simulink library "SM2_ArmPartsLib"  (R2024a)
settings: Solver=ode45  StartTime=0.0  StopTime=10.0  RelTol=1e-3  EnableMultiTasking=on
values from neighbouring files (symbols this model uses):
  m = v*BEAM.rho    [FlexBeamModelConstruct2.m]    (also in FlexBeamModelConstruct3.m = BEAM.rho*v; FlexBeam_1D_Construct.m = REF.m/REF.l*a.*(linspace(1-OPT.MassBiais+1e-6,1+OPT.MassBiai; FlexBeam_3D_Construct.m = REF.m/REF.l*a.*(linspace(1-OPT.MassBiais+1e-6,1+OPT.MassBiai; FreeFlexBeam_3D_Construct.m = REF.m/REF.l*a.*tmp2)
  N = D(1)+(H4^2+H3^2)/H2^2-(E(1)*H4+F(1)*H3)/H2    [MGD.m]    (also in MGD2.m)
  s = -sign(imag(KGZ_fr_tmp))    [LinprogReguliOptimFunc_1.m]    (also in LinprogReguliOptimFunc_2.m; LinprogReguliOptimFunc_1 - Copie.m)
  X = cos(phi(i))*x+sin(phi(i))*y    [MGI.m]
  Y = fft(y(:,i),NFFT)/L    [fft_bis.m]    (also in MGI.m = -sin(phi(i))*x+cos(phi(i))*y)
  Z = z    [MGI.m]
undefined symbols (not defined in the file or in its folder): deg, kg, rad, SimParam
libraries: $bdroot x38, sm_lib x32
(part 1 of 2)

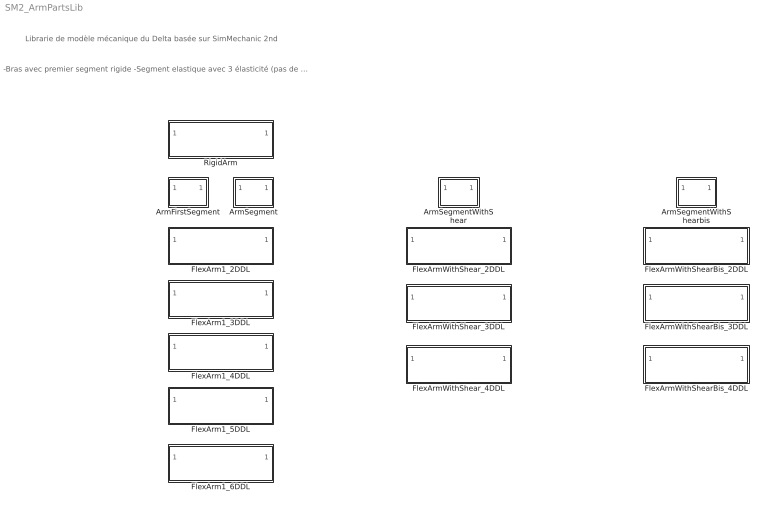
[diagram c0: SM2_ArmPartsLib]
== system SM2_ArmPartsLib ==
  note: -Bras avec premier segment rigide -Segment elastique avec 3 élasticité (pas de cisaillement)
  note: Librarie de modèle mécanique du Delta basée sur SimMechanic 2nd
  ArmFirstSegment : Subsystem  mask{ID=1}
      mask prompts: ID "Segment ID"
  ArmSegment : Subsystem  mask{ID=2}
      mask prompts: ID "Segment ID"
  ArmSegmentWithShear : Subsystem  mask{ID=1}
      mask prompts: ID "Segment ID"
  ArmSegmentWithShearbis : Subsystem  mask{ID=1}
      mask prompts: ID "Segment ID"
  FlexArm1_2DDL : Subsystem  InitFcn=SimParam.Arm = flexArm1_paramInitFnc(RawParam,2,1);  VariantControl=armVarFlex1_2ddl
  FlexArm1_3DDL : Subsystem  InitFcn=SimParam.Arm = flexArm1_paramInitFnc(RawParam,3,1);  VariantControl=armVarFlex1_3ddl
  FlexArm1_4DDL : Subsystem  InitFcn=SimParam.Arm = flexArm1_paramInitFnc(RawParam,4,1);  VariantControl=armVarFlex1_4ddl
  FlexArm1_5DDL : Subsystem  InitFcn=SimParam.Arm = flexArm1_paramInitFnc(RawParam,5,1);  VariantControl=armVarFlex1_4ddl
  FlexArm1_6DDL : Subsystem  InitFcn=SimParam.Arm = flexArm1_paramInitFnc(RawParam,6,1);  VariantControl=armVarFlex1_4ddl
  FlexArmWithShearBis_2DDL : Subsystem  InitFcn=SimParam.Arm = flexArm1_paramInitFnc(RawParam,2,2);  VariantControl=armVarFlex1_2ddl
  FlexArmWithShearBis_3DDL : Subsystem  InitFcn=SimParam.Arm = flexArm1_paramInitFnc(RawParam,3,2);  VariantControl=armVarFlex1_2ddl
  FlexArmWithShearBis_4DDL : Subsystem  InitFcn=SimParam.Arm = flexArm1_paramInitFnc(RawParam,4,2);  VariantControl=armVarFlex1_2ddl
  FlexArmWithShear_2DDL : Subsystem  InitFcn=SimParam.Arm = flexArm1_paramInitFnc(RawParam,2,2);  VariantControl=armVarFlex1_2ddl
  FlexArmWithShear_3DDL : Subsystem  InitFcn=SimParam.Arm = flexArm1_paramInitFnc(RawParam,3,2);  VariantControl=armVarFlex1_2ddl
  FlexArmWithShear_4DDL : Subsystem  InitFcn=SimParam.Arm = flexArm1_paramInitFnc(RawParam,4,2);  VariantControl=armVarFlex1_2ddl
  RigidArm : Subsystem  InitFcn=SimParam.Arm=RigidArm_paramInitFnc(RawParam,0);  VariantControl=armVarDefault

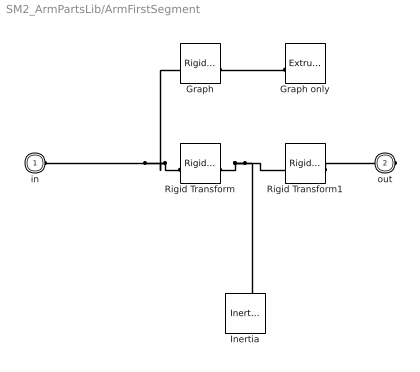
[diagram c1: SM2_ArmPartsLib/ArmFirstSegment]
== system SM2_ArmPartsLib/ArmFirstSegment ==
  Graph : sm_lib/Frames and Transforms/Rigid Transform  RotationMethod=AlignedAxes  FollAlignAxisA=+Z  BaseAlignAxisA=+X  FollAlignAxisB=+Y  BaseAlignAxisB=+Z  RotationStandardAxis=+Z  RotationAngle=0  RotationAngleUnits=deg  RotationArbitraryAxis=[0 0 1]  RotationSequenceAxes=FollowerAxes  RotationSequence=XYX  RotationSequenceAngles=[0 0 0]  RotationSequenceAnglesUnits=deg  RotationMatrix=[1 0 0;0 1 0;0 0 1]  Quaternion=[1 0 0 0]  TranslationMethod=Cartesian  TranslationCartesianOffset=[(SimParam.Arm.l(1,ID)+SimParam.Arm.l(2,ID))/2 0 0]  TranslationCartesianOffsetUnits=m  TranslationStandardAxis=+Z  TranslationStandardOffset=0  TranslationStandardOffsetUnits=m  TranslationROffset=0  TranslationROffsetUnits=m  TranslationThetaOffset=0  TranslationThetaOffsetUnits=deg  TranslationZOffset=0  TranslationZOffsetUnits=m
  Graph only : sm_lib/Body Elements/Extruded Solid  ExtrusionType=General  PolygonNumSides=3  PolygonOuterRadius=1  PolygonOuterRadiusUnits=m  ExportEntireGeometry=off  ExtrusionCrossSection=0.01.*[1 1; -1 1; -1 -1; 1 -1]  ExtrusionCrossSectionUnits=m  ExportConvexHullGeometry=off  ExtrusionLength=SimParam.Arm.l(1,ID)+SimParam.Arm.l(2,ID)  ExtrusionLengthUnits=m  InertiaType=PointMass  BasedOnType=Density  Density=1000  DensityUnits=kg/(m^3)  Mass=0  MassUnits=kg  CenterOfMass=[0 0 0]  CenterOfMassUnits=m  MomentsOfInertia=[0 0 0]  MomentsOfInertiaUnits=kg*m^2  ProductsOfInertia=[0 0 0]  ProductsOfInertiaUnits=kg*m^2  GraphicType=FromGeometry  MarkerShape=Sphere  MarkerSize=10  GraphicVisPropType=SimpleVisualProperties  GraphicDiffuseColor=[0.5 0.5 0.5]  GraphicOpacity=1.0  GraphicSpecularColor=[0.5 0.5 0.5 1.0]  GraphicAmbientColor=[0.15 0.15 0.15 1.0]  GraphicEmissiveColor=[0.0 0.0 0.0 1.0]  GraphicShininess=75  DoExposeReferenceFrame=on  SerializedFrames=<Frames/>
  Inertia : sm_lib/Body Elements/Inertia  InertiaType=Custom  Mass=SimParam.Arm.m(ID)  MassUnits=kg  CenterOfMass=[0 0 0]  CenterOfMassUnits=m  MomentsOfInertia=SimParam.Arm.I(:,ID)'  MomentsOfInertiaUnits=kg*m^2  ProductsOfInertia=[0 0 0]  ProductsOfInertiaUnits=kg*m^2  GraphicType=Marker  MarkerShape=Inertia  MarkerSize=20  GraphicVisPropType=SimpleVisualProperties  GraphicDiffuseColor=[0.5 0.5 0.5]  GraphicOpacity=1  GraphicSpecularColor=[0.5 0.5 0.5 1.0]  GraphicAmbientColor=[0.15 0.15 0.15 1.0]  GraphicEmissiveColor=[0.0 0.0 0.0 1.0]  GraphicShininess=75
  Rigid Transform : sm_lib/Frames and Transforms/Rigid Transform  RotationMethod=None  FollAlignAxisA=+X  BaseAlignAxisA=+Y  FollAlignAxisB=+Y  BaseAlignAxisB=+Z  RotationStandardAxis=+Z  RotationAngle=0  RotationAngleUnits=deg  RotationArbitraryAxis=[0 0 1]  RotationSequenceAxes=FollowerAxes  RotationSequence=XYX  RotationSequenceAngles=[0 0 0]  RotationSequenceAnglesUnits=deg  RotationMatrix=[1 0 0;0 1 0;0 0 1]  Quaternion=[1 0 0 0]  TranslationMethod=Cartesian  TranslationCartesianOffset=[SimParam.Arm.l(1,ID) 0 0]  TranslationCartesianOffsetUnits=m  TranslationStandardAxis=+Z  TranslationStandardOffset=0  TranslationStandardOffsetUnits=m  TranslationROffset=0  TranslationROffsetUnits=m  TranslationThetaOffset=0  TranslationThetaOffsetUnits=deg  TranslationZOffset=0  TranslationZOffsetUnits=m
  Rigid Transform1 : sm_lib/Frames and Transforms/Rigid Transform  RotationMethod=None  FollAlignAxisA=+X  BaseAlignAxisA=+Y  FollAlignAxisB=+Y  BaseAlignAxisB=+Z  RotationStandardAxis=+Z  RotationAngle=0  RotationAngleUnits=deg  RotationArbitraryAxis=[0 0 1]  RotationSequenceAxes=FollowerAxes  RotationSequence=XYX  RotationSequenceAngles=[0 0 0]  RotationSequenceAnglesUnits=deg  RotationMatrix=[1 0 0;0 1 0;0 0 1]  Quaternion=[1 0 0 0]  TranslationMethod=Cartesian  TranslationCartesianOffset=[SimParam.Arm.l(2,ID) 0 0]  TranslationCartesianOffsetUnits=m  TranslationStandardAxis=+Z  TranslationStandardOffset=0  TranslationStandardOffsetUnits=m  TranslationROffset=0  TranslationROffsetUnits=m  TranslationThetaOffset=0  TranslationThetaOffsetUnits=deg  TranslationZOffset=0  TranslationZOffsetUnits=m
  in : PMIOPort  Side=Left
  out : PMIOPort  Port=2  Side=Right
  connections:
  Rigid Transform/RConn1 -- Rigid Transform1/LConn1 -- Inertia/RConn1
  Rigid Transform1/RConn1 -- out/RConn1
  Rigid Transform/LConn1 -- in/RConn1 -- Graph/LConn1
  Graph only/RConn1 -- Graph/RConn1

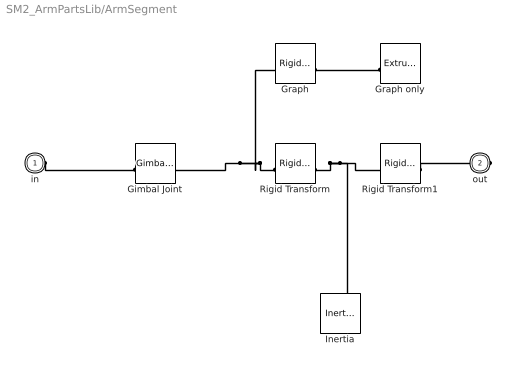
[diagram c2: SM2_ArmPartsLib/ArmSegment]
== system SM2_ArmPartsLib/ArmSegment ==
  Gimbal Joint : sm_lib/Joints/Gimbal Joint  JointMode=Normal  CompositeWrenchDir=FollowerOnBase  CompositeWrenchFrame=BaseFrame  SenseConstraintForce=off  SenseConstraintTorque=off  SenseTotalForce=off  SenseTotalTorque=off  RxPositionTargetSpecify=on  RxPositionTargetPriority=High  RxPositionTargetValue=0  RxPositionTargetValueUnits=rad  RxVelocityTargetSpecify=on  RxVelocityTargetPriority=High  RxVelocityTargetValue=0  RxVelocityTargetValueUnits=rad/s  RxEquilibriumPosition=0  RxEquilibriumPositionUnits=rad  RxSpringStiffness=SimParam.Arm.k(1,ID)  RxSpringStiffnessUnits=N*m/rad  RxDampingCoefficient=SimParam.Arm.c(1,ID)  RxDampingCoefficientUnits=N*m/(rad/s)  RxLowerLimitSpecify=off  RxLowerLimitBound=-90  RxLowerLimitBoundUnits=deg  RxLowerLimitStiffness=1e4  RxLowerLimitStiffnessUnits=N*m/deg  RxLowerLimitDamping=10  RxLowerLimitDampingUnits=N*m/(deg/s)  RxLowerLimitTransitionRegionWidth=0.1  RxLowerLimitTransitionRegionWidthUnits=deg  RxUpperLimitSpecify=off  RxUpperLimitBound=90  RxUpperLimitBoundUnits=deg  RxUpperLimitStiffness=1e4  RxUpperLimitStiffnessUnits=N*m/deg  RxUpperLimitDamping=10  RxUpperLimitDampingUnits=N*m/(deg/s)  RxUpperLimitTransitionRegionWidth=0.1  RxUpperLimitTransitionRegionWidthUnits=deg  RxTorqueActuationMode=NoTorque  RxMotionActuationMode=ComputedMotion  RxSensePosition=off  RxSenseVelocity=off  RxSenseAcceleration=off  RxSenseTorqueForce=off  RxSenseLowerLimitTorqueForce=off  RxSenseUpperLimitTorqueForce=off  RyPositionTargetSpecify=on  RyPositionTargetPriority=High  RyPositionTargetValue=0  RyPositionTargetValueUnits=rad  RyVelocityTargetSpecify=on  RyVelocityTargetPriority=High  RyVelocityTargetValue=0  RyVelocityTargetValueUnits=rad/s  RyEquilibriumPosition=0  RyEquilibriumPositionUnits=rad  RySpringStiffness=SimParam.Arm.k(2,ID)  RySpringStiffnessUnits=N*m/rad  RyDampingCoefficient=SimParam.Arm.c(2,ID)  RyDampingCoefficientUnits=N*m/(rad/s)  RyLowerLimitSpecify=off  RyLowerLimitBound=-90  RyLowerLimitBoundUnits=deg  RyLowerLimitStiffness=1e4  RyLowerLimitStiffnessUnits=N*m/deg  RyLowerLimitDamping=10  RyLowerLimitDampingUnits=N*m/(deg/s)  RyLowerLimitTransitionRegionWidth=0.1  RyLowerLimitTransitionRegionWidthUnits=deg  RyUpperLimitSpecify=off  RyUpperLimitBound=90  RyUpperLimitBoundUnits=deg  RyUpperLimitStiffness=1e4  RyUpperLimitStiffnessUnits=N*m/deg  RyUpperLimitDamping=10  RyUpperLimitDampingUnits=N*m/(deg/s)  RyUpperLimitTransitionRegionWidth=0.1  RyUpperLimitTransitionRegionWidthUnits=deg  RyTorqueActuationMode=NoTorque  RyMotionActuationMode=ComputedMotion  RySensePosition=off  RySenseVelocity=off  RySenseAcceleration=off  RySenseTorqueForce=off  RySenseLowerLimitTorqueForce=off  RySenseUpperLimitTorqueForce=off  RzPositionTargetSpecify=on  RzPositionTargetPriority=High  RzPositionTargetValue=0  RzPositionTargetValueUnits=rad  RzVelocityTargetSpecify=on  RzVelocityTargetPriority=High  RzVelocityTargetValue=0  RzVelocityTargetValueUnits=rad/s  RzEquilibriumPosition=0  RzEquilibriumPositionUnits=rad  RzSpringStiffness=SimParam.Arm.k(3,ID)  RzSpringStiffnessUnits=N*m/rad  RzDampingCoefficient=SimParam.Arm.c(3,ID)  RzDampingCoefficientUnits=N*m/(rad/s)  RzLowerLimitSpecify=off  RzLowerLimitBound=-90  RzLowerLimitBoundUnits=deg  RzLowerLimitStiffness=1e4  RzLowerLimitStiffnessUnits=N*m/deg  RzLowerLimitDamping=10  RzLowerLimitDampingUnits=N*m/(deg/s)  RzLowerLimitTransitionRegionWidth=0.1  RzLowerLimitTransitionRegionWidthUnits=deg  RzUpperLimitSpecify=off  RzUpperLimitBound=90  RzUpperLimitBoundUnits=deg  RzUpperLimitStiffness=1e4  RzUpperLimitStiffnessUnits=N*m/deg  RzUpperLimitDamping=10  RzUpperLimitDampingUnits=N*m/(deg/s)  RzUpperLimitTransitionRegionWidth=0.1  RzUpperLimitTransitionRegionWidthUnits=deg  RzTorqueActuationMode=NoTorque  RzMotionActuationMode=ComputedMotion  RzSensePosition=off  RzSenseVelocity=off  RzSenseAcceleration=off  RzSenseTorqueForce=off  RzSenseLowerLimitTorqueForce=off  RzSenseUpperLimitTorqueForce=off
  Graph : sm_lib/Frames and Transforms/Rigid Transform  RotationMethod=AlignedAxes  FollAlignAxisA=+Z  BaseAlignAxisA=+X  FollAlignAxisB=+Y  BaseAlignAxisB=+Z  RotationStandardAxis=+Z  RotationAngle=0  RotationAngleUnits=deg  RotationArbitraryAxis=[0 0 1]  RotationSequenceAxes=FollowerAxes  RotationSequence=XYX  RotationSequenceAngles=[0 0 0]  RotationSequenceAnglesUnits=deg  RotationMatrix=[1 0 0;0 1 0;0 0 1]  Quaternion=[1 0 0 0]  TranslationMethod=Cartesian  TranslationCartesianOffset=[(SimParam.Arm.l(1,ID)+SimParam.Arm.l(2,ID))/2 0 0]  TranslationCartesianOffsetUnits=m  TranslationStandardAxis=+Z  TranslationStandardOffset=0  TranslationStandardOffsetUnits=m  TranslationROffset=0  TranslationROffsetUnits=m  TranslationThetaOffset=0  TranslationThetaOffsetUnits=deg  TranslationZOffset=0  TranslationZOffsetUnits=m
  Graph only : sm_lib/Body Elements/Extruded Solid  ExtrusionType=General  PolygonNumSides=3  PolygonOuterRadius=1  PolygonOuterRadiusUnits=m  ExportEntireGeometry=off  ExtrusionCrossSection=0.01.*[1 1; -1 1; -1 -1; 1 -1]  ExtrusionCrossSectionUnits=m  ExportConvexHullGeometry=off  ExtrusionLength=SimParam.Arm.l(1,ID)+SimParam.Arm.l(2,ID)  ExtrusionLengthUnits=m  InertiaType=PointMass  BasedOnType=Density  Density=1000  DensityUnits=kg/(m^3)  Mass=0  MassUnits=kg  CenterOfMass=[0 0 0]  CenterOfMassUnits=m  MomentsOfInertia=[0 0 0]  MomentsOfInertiaUnits=kg*m^2  ProductsOfInertia=[0 0 0]  ProductsOfInertiaUnits=kg*m^2  GraphicType=FromGeometry  MarkerShape=Sphere  MarkerSize=10  GraphicVisPropType=SimpleVisualProperties  GraphicDiffuseColor=[0.5 0.5 0.5]  GraphicOpacity=1.0  GraphicSpecularColor=[0.5 0.5 0.5 1.0]  GraphicAmbientColor=[0.15 0.15 0.15 1.0]  GraphicEmissiveColor=[0.0 0.0 0.0 1.0]  GraphicShininess=75  DoExposeReferenceFrame=on  SerializedFrames=<Frames/>
  Inertia : sm_lib/Body Elements/Inertia  InertiaType=Custom  Mass=SimParam.Arm.m(ID)  MassUnits=kg  CenterOfMass=[0 0 0]  CenterOfMassUnits=m  MomentsOfInertia=SimParam.Arm.I(:,ID)'  MomentsOfInertiaUnits=kg*m^2  ProductsOfInertia=[0 0 0]  ProductsOfInertiaUnits=kg*m^2  GraphicType=Marker  MarkerShape=Inertia  MarkerSize=20  GraphicVisPropType=SimpleVisualProperties  GraphicDiffuseColor=[0.5 0.5 0.5]  GraphicOpacity=1  GraphicSpecularColor=[0.5 0.5 0.5 1.0]  GraphicAmbientColor=[0.15 0.15 0.15 1.0]  GraphicEmissiveColor=[0.0 0.0 0.0 1.0]  GraphicShininess=75
  Rigid Transform : sm_lib/Frames and Transforms/Rigid Transform  RotationMethod=None  FollAlignAxisA=+X  BaseAlignAxisA=+Y  FollAlignAxisB=+Y  BaseAlignAxisB=+Z  RotationStandardAxis=+Z  RotationAngle=0  RotationAngleUnits=deg  RotationArbitraryAxis=[0 0 1]  RotationSequenceAxes=FollowerAxes  RotationSequence=XYX  RotationSequenceAngles=[0 0 0]  RotationSequenceAnglesUnits=deg  RotationMatrix=[1 0 0;0 1 0;0 0 1]  Quaternion=[1 0 0 0]  TranslationMethod=Cartesian  TranslationCartesianOffset=[SimParam.Arm.l(1,ID) 0 0]  TranslationCartesianOffsetUnits=m  TranslationStandardAxis=+Z  TranslationStandardOffset=0  TranslationStandardOffsetUnits=m  TranslationROffset=0  TranslationROffsetUnits=m  TranslationThetaOffset=0  TranslationThetaOffsetUnits=deg  TranslationZOffset=0  TranslationZOffsetUnits=m
  Rigid Transform1 : sm_lib/Frames and Transforms/Rigid Transform  RotationMethod=None  FollAlignAxisA=+X  BaseAlignAxisA=+Y  FollAlignAxisB=+Y  BaseAlignAxisB=+Z  RotationStandardAxis=+Z  RotationAngle=0  RotationAngleUnits=deg  RotationArbitraryAxis=[0 0 1]  RotationSequenceAxes=FollowerAxes  RotationSequence=XYX  RotationSequenceAngles=[0 0 0]  RotationSequenceAnglesUnits=deg  RotationMatrix=[1 0 0;0 1 0;0 0 1]  Quaternion=[1 0 0 0]  TranslationMethod=Cartesian  TranslationCartesianOffset=[SimParam.Arm.l(2,ID) 0 0]  TranslationCartesianOffsetUnits=m  TranslationStandardAxis=+Z  TranslationStandardOffset=0  TranslationStandardOffsetUnits=m  TranslationROffset=0  TranslationROffsetUnits=m  TranslationThetaOffset=0  TranslationThetaOffsetUnits=deg  TranslationZOffset=0  TranslationZOffsetUnits=m
  in : PMIOPort  Side=Left
  out : PMIOPort  Port=2  Side=Right
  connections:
  Rigid Transform/RConn1 -- Rigid Transform1/LConn1 -- Inertia/RConn1
  Rigid Transform/LConn1 -- Gimbal Joint/RConn1 -- Graph/LConn1
  Rigid Transform1/RConn1 -- out/RConn1
  in/RConn1 -- Gimbal Joint/LConn1
  Graph only/RConn1 -- Graph/RConn1

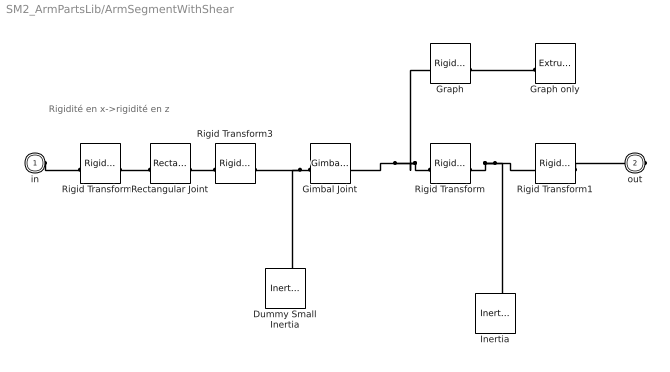
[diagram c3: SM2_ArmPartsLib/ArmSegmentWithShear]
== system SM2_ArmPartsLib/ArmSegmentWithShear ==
  note: Rigidité en x->rigidité en z
  Dummy Small Inertia : sm_lib/Body Elements/Inertia  InertiaType=Custom  Mass=1e-3*SimParam.Arm.m(ID)  MassUnits=kg  CenterOfMass=[0 0 0]  CenterOfMassUnits=m  MomentsOfInertia=1e-4*SimParam.Arm.I(:,ID)'  MomentsOfInertiaUnits=kg*m^2  ProductsOfInertia=[0 0 0]  ProductsOfInertiaUnits=kg*m^2  GraphicType=Marker  MarkerShape=Inertia  MarkerSize=20  GraphicVisPropType=SimpleVisualProperties  GraphicDiffuseColor=[0.5 0.5 0.5]  GraphicOpacity=1  GraphicSpecularColor=[0.5 0.5 0.5 1.0]  GraphicAmbientColor=[0.15 0.15 0.15 1.0]  GraphicEmissiveColor=[0.0 0.0 0.0 1.0]  GraphicShininess=75
  Gimbal Joint : sm_lib/Joints/Gimbal Joint  JointMode=Normal  CompositeWrenchDir=FollowerOnBase  CompositeWrenchFrame=BaseFrame  SenseConstraintForce=off  SenseConstraintTorque=off  SenseTotalForce=off  SenseTotalTorque=off  RxPositionTargetSpecify=on  RxPositionTargetPriority=High  RxPositionTargetValue=0  RxPositionTargetValueUnits=rad  RxVelocityTargetSpecify=on  RxVelocityTargetPriority=High  RxVelocityTargetValue=0  RxVelocityTargetValueUnits=rad/s  RxEquilibriumPosition=0  RxEquilibriumPositionUnits=rad  RxSpringStiffness=SimParam.Arm.k(4,ID)  RxSpringStiffnessUnits=N*m/rad  RxDampingCoefficient=SimParam.Arm.c(4,ID)  RxDampingCoefficientUnits=N*m/(rad/s)  RxLowerLimitSpecify=off  RxLowerLimitBound=-90  RxLowerLimitBoundUnits=deg  RxLowerLimitStiffness=1e4  RxLowerLimitStiffnessUnits=N*m/deg  RxLowerLimitDamping=10  RxLowerLimitDampingUnits=N*m/(deg/s)  RxLowerLimitTransitionRegionWidth=0.1  RxLowerLimitTransitionRegionWidthUnits=deg  RxUpperLimitSpecify=off  RxUpperLimitBound=90  RxUpperLimitBoundUnits=deg  RxUpperLimitStiffness=1e4  RxUpperLimitStiffnessUnits=N*m/deg  RxUpperLimitDamping=10  RxUpperLimitDampingUnits=N*m/(deg/s)  RxUpperLimitTransitionRegionWidth=0.1  RxUpperLimitTransitionRegionWidthUnits=deg  RxTorqueActuationMode=NoTorque  RxMotionActuationMode=ComputedMotion  RxSensePosition=off  RxSenseVelocity=off  RxSenseAcceleration=off  RxSenseTorqueForce=off  RxSenseLowerLimitTorqueForce=off  RxSenseUpperLimitTorqueForce=off  RyPositionTargetSpecify=on  RyPositionTargetPriority=High  RyPositionTargetValue=0  RyPositionTargetValueUnits=rad  RyVelocityTargetSpecify=on  RyVelocityTargetPriority=High  RyVelocityTargetValue=0  RyVelocityTargetValueUnits=rad/s  RyEquilibriumPosition=0  RyEquilibriumPositionUnits=rad  RySpringStiffness=SimParam.Arm.k(5,ID)  RySpringStiffnessUnits=N*m/rad  RyDampingCoefficient=SimParam.Arm.c(5,ID)  RyDampingCoefficientUnits=N*m/(rad/s)  RyLowerLimitSpecify=off  RyLowerLimitBound=-90  RyLowerLimitBoundUnits=deg  RyLowerLimitStiffness=1e4  RyLowerLimitStiffnessUnits=N*m/deg  RyLowerLimitDamping=10  RyLowerLimitDampingUnits=N*m/(deg/s)  RyLowerLimitTransitionRegionWidth=0.1  RyLowerLimitTransitionRegionWidthUnits=deg  RyUpperLimitSpecify=off  RyUpperLimitBound=90  RyUpperLimitBoundUnits=deg  RyUpperLimitStiffness=1e4  RyUpperLimitStiffnessUnits=N*m/deg  RyUpperLimitDamping=10  RyUpperLimitDampingUnits=N*m/(deg/s)  RyUpperLimitTransitionRegionWidth=0.1  RyUpperLimitTransitionRegionWidthUnits=deg  RyTorqueActuationMode=NoTorque  RyMotionActuationMode=ComputedMotion  RySensePosition=off  RySenseVelocity=off  RySenseAcceleration=off  RySenseTorqueForce=off  RySenseLowerLimitTorqueForce=off  RySenseUpperLimitTorqueForce=off  RzPositionTargetSpecify=on  RzPositionTargetPriority=High  RzPositionTargetValue=0  RzPositionTargetValueUnits=rad  RzVelocityTargetSpecify=on  RzVelocityTargetPriority=High  RzVelocityTargetValue=0  RzVelocityTargetValueUnits=rad/s  RzEquilibriumPosition=0  RzEquilibriumPositionUnits=rad  RzSpringStiffness=SimParam.Arm.k(6,ID)  RzSpringStiffnessUnits=N*m/rad  RzDampingCoefficient=SimParam.Arm.c(6,ID)  RzDampingCoefficientUnits=N*m/(rad/s)  RzLowerLimitSpecify=off  RzLowerLimitBound=-90  RzLowerLimitBoundUnits=deg  RzLowerLimitStiffness=1e4  RzLowerLimitStiffnessUnits=N*m/deg  RzLowerLimitDamping=10  RzLowerLimitDampingUnits=N*m/(deg/s)  RzLowerLimitTransitionRegionWidth=0.1  RzLowerLimitTransitionRegionWidthUnits=deg  RzUpperLimitSpecify=off  RzUpperLimitBound=90  RzUpperLimitBoundUnits=deg  RzUpperLimitStiffness=1e4  RzUpperLimitStiffnessUnits=N*m/deg  RzUpperLimitDamping=10  RzUpperLimitDampingUnits=N*m/(deg/s)  RzUpperLimitTransitionRegionWidth=0.1  RzUpperLimitTransitionRegionWidthUnits=deg  RzTorqueActuationMode=NoTorque  RzMotionActuationMode=ComputedMotion  RzSensePosition=off  RzSenseVelocity=off  RzSenseAcceleration=off  RzSenseTorqueForce=off  RzSenseLowerLimitTorqueForce=off  RzSenseUpperLimitTorqueForce=off
  Graph : sm_lib/Frames and Transforms/Rigid Transform  RotationMethod=AlignedAxes  FollAlignAxisA=+Z  BaseAlignAxisA=+X  FollAlignAxisB=+Y  BaseAlignAxisB=+Z  RotationStandardAxis=+Z  RotationAngle=0  RotationAngleUnits=deg  RotationArbitraryAxis=[0 0 1]  RotationSequenceAxes=FollowerAxes  RotationSequence=XYX  RotationSequenceAngles=[0 0 0]  RotationSequenceAnglesUnits=deg  RotationMatrix=[1 0 0;0 1 0;0 0 1]  Quaternion=[1 0 0 0]  TranslationMethod=Cartesian  TranslationCartesianOffset=[(SimParam.Arm.l(1,ID)+SimParam.Arm.l(2,ID))/2 0 0]  TranslationCartesianOffsetUnits=m  TranslationStandardAxis=+Z  TranslationStandardOffset=0  TranslationStandardOffsetUnits=m  TranslationROffset=0  TranslationROffsetUnits=m  TranslationThetaOffset=0  TranslationThetaOffsetUnits=deg  TranslationZOffset=0  TranslationZOffsetUnits=m
  Graph only : sm_lib/Body Elements/Extruded Solid  ExtrusionType=General  PolygonNumSides=3  PolygonOuterRadius=1  PolygonOuterRadiusUnits=m  ExportEntireGeometry=off  ExtrusionCrossSection=0.01.*[1 1; -1 1; -1 -1; 1 -1]  ExtrusionCrossSectionUnits=m  ExportConvexHullGeometry=off  ExtrusionLength=SimParam.Arm.l(1,ID)+SimParam.Arm.l(2,ID)  ExtrusionLengthUnits=m  InertiaType=PointMass  BasedOnType=Density  Density=1000  DensityUnits=kg/(m^3)  Mass=0  MassUnits=kg  CenterOfMass=[0 0 0]  CenterOfMassUnits=m  MomentsOfInertia=[0 0 0]  MomentsOfInertiaUnits=kg*m^2  ProductsOfInertia=[0 0 0]  ProductsOfInertiaUnits=kg*m^2  GraphicType=FromGeometry  MarkerShape=Sphere  MarkerSize=10  GraphicVisPropType=SimpleVisualProperties  GraphicDiffuseColor=[0.5 0.5 0.5]  GraphicOpacity=1.0  GraphicSpecularColor=[0.5 0.5 0.5 1.0]  GraphicAmbientColor=[0.15 0.15 0.15 1.0]  GraphicEmissiveColor=[0.0 0.0 0.0 1.0]  GraphicShininess=75  DoExposeReferenceFrame=on  SerializedFrames=<Frames/>
  Inertia : sm_lib/Body Elements/Inertia  InertiaType=Custom  Mass=SimParam.Arm.m(ID)  MassUnits=kg  CenterOfMass=[0 0 0]  CenterOfMassUnits=m  MomentsOfInertia=SimParam.Arm.I(:,ID)'  MomentsOfInertiaUnits=kg*m^2  ProductsOfInertia=[0 0 0]  ProductsOfInertiaUnits=kg*m^2  GraphicType=Marker  MarkerShape=Inertia  MarkerSize=20  GraphicVisPropType=SimpleVisualProperties  GraphicDiffuseColor=[0.5 0.5 0.5]  GraphicOpacity=1  GraphicSpecularColor=[0.5 0.5 0.5 1.0]  GraphicAmbientColor=[0.15 0.15 0.15 1.0]  GraphicEmissiveColor=[0.0 0.0 0.0 1.0]  GraphicShininess=75
  Rectangular Joint : sm_lib/Joints/Rectangular Joint  JointMode=Normal  CompositeWrenchDir=FollowerOnBase  CompositeWrenchFrame=BaseFrame  SenseConstraintForce=off  SenseConstraintTorque=off  SenseTotalForce=off  SenseTotalTorque=off  PxPositionTargetSpecify=on  PxPositionTargetPriority=High  PxPositionTargetValue=0  PxPositionTargetValueUnits=m  PxVelocityTargetSpecify=on  PxVelocityTargetPriority=High  PxVelocityTargetValue=0  PxVelocityTargetValueUnits=m/s  PxEquilibriumPosition=0  PxEquilibriumPositionUnits=m  PxSpringStiffness=SimParam.Arm.k(3,ID)  PxSpringStiffnessUnits=N/m  PxDampingCoefficient=SimParam.Arm.c(3,ID)  PxDampingCoefficientUnits=N/(m/s)  PxLowerLimitSpecify=off  PxLowerLimitBound=-1  PxLowerLimitBoundUnits=m  PxLowerLimitStiffness=1e6  PxLowerLimitStiffnessUnits=N/m  PxLowerLimitDamping=1e3  PxLowerLimitDampingUnits=N/(m/s)  PxLowerLimitTransitionRegionWidth=1e-4  PxLowerLimitTransitionRegionWidthUnits=m  PxUpperLimitSpecify=off  PxUpperLimitBound=1  PxUpperLimitBoundUnits=m  PxUpperLimitStiffness=1e6  PxUpperLimitStiffnessUnits=N/m  PxUpperLimitDamping=1e3  PxUpperLimitDampingUnits=N/(m/s)  PxUpperLimitTransitionRegionWidth=1e-4  PxUpperLimitTransitionRegionWidthUnits=m  PxTorqueActuationMode=NoTorque  PxMotionActuationMode=ComputedMotion  PxSensePosition=off  PxSenseVelocity=off  PxSenseAcceleration=off  PxSenseTorqueForce=off  PxSenseLowerLimitTorqueForce=off  PxSenseUpperLimitTorqueForce=off  PyPositionTargetSpecify=on  PyPositionTargetPriority=High  PyPositionTargetValue=0  PyPositionTargetValueUnits=m  PyVelocityTargetSpecify=on  PyVelocityTargetPriority=High  PyVelocityTargetValue=0  PyVelocityTargetValueUnits=m/s  PyEquilibriumPosition=0  PyEquilibriumPositionUnits=m  PySpringStiffness=SimParam.Arm.k(2,ID)  PySpringStiffnessUnits=N/m  PyDampingCoefficient=SimParam.Arm.c(2,ID)  PyDampingCoefficientUnits=N/(m/s)  PyLowerLimitSpecify=off  PyLowerLimitBound=-1  PyLowerLimitBoundUnits=m  PyLowerLimitStiffness=1e6  PyLowerLimitStiffnessUnits=N/m  PyLowerLimitDamping=1e3  PyLowerLimitDampingUnits=N/(m/s)  PyLowerLimitTransitionRegionWidth=1e-4  PyLowerLimitTransitionRegionWidthUnits=m  PyUpperLimitSpecify=off  PyUpperLimitBound=1  PyUpperLimitBoundUnits=m  PyUpperLimitStiffness=1e6  PyUpperLimitStiffnessUnits=N/m  PyUpperLimitDamping=1e3  PyUpperLimitDampingUnits=N/(m/s)  PyUpperLimitTransitionRegionWidth=1e-4  PyUpperLimitTransitionRegionWidthUnits=m  PyTorqueActuationMode=NoTorque  PyMotionActuationMode=ComputedMotion  PySensePosition=off  PySenseVelocity=off  PySenseAcceleration=off  PySenseTorqueForce=off  PySenseLowerLimitTorqueForce=off  PySenseUpperLimitTorqueForce=off
  Rigid Transform : sm_lib/Frames and Transforms/Rigid Transform  RotationMethod=None  FollAlignAxisA=+X  BaseAlignAxisA=+Y  FollAlignAxisB=+Y  BaseAlignAxisB=+Z  RotationStandardAxis=+Z  RotationAngle=0  RotationAngleUnits=deg  RotationArbitraryAxis=[0 0 1]  RotationSequenceAxes=FollowerAxes  RotationSequence=XYX  RotationSequenceAngles=[0 0 0]  RotationSequenceAnglesUnits=deg  RotationMatrix=[1 0 0;0 1 0;0 0 1]  Quaternion=[1 0 0 0]  TranslationMethod=Cartesian  TranslationCartesianOffset=[SimParam.Arm.l(1,ID) 0 0]  TranslationCartesianOffsetUnits=m  TranslationStandardAxis=+Z  TranslationStandardOffset=0  TranslationStandardOffsetUnits=m  TranslationROffset=0  TranslationROffsetUnits=m  TranslationThetaOffset=0  TranslationThetaOffsetUnits=deg  TranslationZOffset=0  TranslationZOffsetUnits=m
  Rigid Transform1 : sm_lib/Frames and Transforms/Rigid Transform  RotationMethod=None  FollAlignAxisA=+X  BaseAlignAxisA=+Y  FollAlignAxisB=+Y  BaseAlignAxisB=+Z  RotationStandardAxis=+Z  RotationAngle=0  RotationAngleUnits=deg  RotationArbitraryAxis=[0 0 1]  RotationSequenceAxes=FollowerAxes  RotationSequence=XYX  RotationSequenceAngles=[0 0 0]  RotationSequenceAnglesUnits=deg  RotationMatrix=[1 0 0;0 1 0;0 0 1]  Quaternion=[1 0 0 0]  TranslationMethod=Cartesian  TranslationCartesianOffset=[SimParam.Arm.l(2,ID) 0 0]  TranslationCartesianOffsetUnits=m  TranslationStandardAxis=+Z  TranslationStandardOffset=0  TranslationStandardOffsetUnits=m  TranslationROffset=0  TranslationROffsetUnits=m  TranslationThetaOffset=0  TranslationThetaOffsetUnits=deg  TranslationZOffset=0  TranslationZOffsetUnits=m
  Rigid Transform2 : sm_lib/Frames and Transforms/Rigid Transform  RotationMethod=AlignedAxes  FollAlignAxisA=+Z  BaseAlignAxisA=+X  FollAlignAxisB=+Y  BaseAlignAxisB=+Y  RotationStandardAxis=+Z  RotationAngle=0  RotationAngleUnits=deg  RotationArbitraryAxis=[0 0 1]  RotationSequenceAxes=FollowerAxes  RotationSequence=XYX  RotationSequenceAngles=[0 0 0]  RotationSequenceAnglesUnits=deg  RotationMatrix=[1 0 0;0 1 0;0 0 1]  Quaternion=[1 0 0 0]  TranslationMethod=None  TranslationCartesianOffset=[0 0 0]  TranslationCartesianOffsetUnits=m  TranslationStandardAxis=+Z  TranslationStandardOffset=0  TranslationStandardOffsetUnits=m  TranslationROffset=0  TranslationROffsetUnits=m  TranslationThetaOffset=0  TranslationThetaOffsetUnits=deg  TranslationZOffset=0  TranslationZOffsetUnits=m
  Rigid Transform3 : sm_lib/Frames and Transforms/Rigid Transform  RotationMethod=AlignedAxes  FollAlignAxisA=+X  BaseAlignAxisA=+Z  FollAlignAxisB=+Y  BaseAlignAxisB=+Y  RotationStandardAxis=+Z  RotationAngle=0  RotationAngleUnits=deg  RotationArbitraryAxis=[0 0 1]  RotationSequenceAxes=FollowerAxes  RotationSequence=XYX  RotationSequenceAngles=[0 0 0]  RotationSequenceAnglesUnits=deg  RotationMatrix=[1 0 0;0 1 0;0 0 1]  Quaternion=[1 0 0 0]  TranslationMethod=None  TranslationCartesianOffset=[0 0 0]  TranslationCartesianOffsetUnits=m  TranslationStandardAxis=+Z  TranslationStandardOffset=0  TranslationStandardOffsetUnits=m  TranslationROffset=0  TranslationROffsetUnits=m  TranslationThetaOffset=0  TranslationThetaOffsetUnits=deg  TranslationZOffset=0  TranslationZOffsetUnits=m
  in : PMIOPort  Side=Left
  out : PMIOPort  Port=2  Side=Right
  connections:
  Rigid Transform/RConn1 -- Rigid Transform1/LConn1 -- Inertia/RConn1
  Rigid Transform/LConn1 -- Gimbal Joint/RConn1 -- Graph/LConn1
  Rigid Transform1/RConn1 -- out/RConn1
  Graph only/RConn1 -- Graph/RConn1
  in/RConn1 -- Rigid Transform2/LConn1
  Rigid Transform2/RConn1 -- Rectangular Joint/LConn1
  Gimbal Joint/LConn1 -- Dummy Small Inertia/RConn1 -- Rigid Transform3/RConn1
  Rigid Transform3/LConn1 -- Rectangular Joint/RConn1

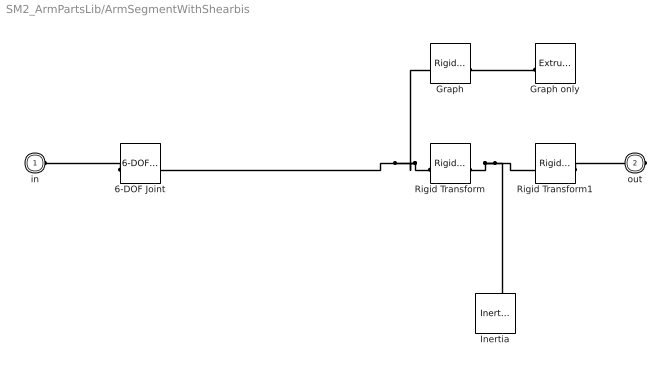
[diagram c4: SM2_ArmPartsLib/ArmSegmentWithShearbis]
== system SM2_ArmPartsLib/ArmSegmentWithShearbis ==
  6-DOF Joint : sm_lib/Joints/6-DOF Joint  JointMode=Normal  CompositeWrenchDir=FollowerOnBase  CompositeWrenchFrame=BaseFrame  SenseConstraintForce=off  SenseConstraintTorque=off  SenseTotalForce=off  SenseTotalTorque=off  PxPositionTargetSpecify=on  PxPositionTargetPriority=High  PxPositionTargetValue=0  PxPositionTargetValueUnits=m  PxVelocityTargetSpecify=on  PxVelocityTargetPriority=High  PxVelocityTargetValue=0  PxVelocityTargetValueUnits=m/s  PxEquilibriumPosition=0  PxEquilibriumPositionUnits=m  PxSpringStiffness=1e13  PxSpringStiffnessUnits=N/m  PxDampingCoefficient=1e10  PxDampingCoefficientUnits=N/(m/s)  PxLowerLimitSpecify=off  PxLowerLimitBound=-1  PxLowerLimitBoundUnits=m  PxLowerLimitStiffness=1e6  PxLowerLimitStiffnessUnits=N/m  PxLowerLimitDamping=1e3  PxLowerLimitDampingUnits=N/(m/s)  PxLowerLimitTransitionRegionWidth=1e-4  PxLowerLimitTransitionRegionWidthUnits=m  PxUpperLimitSpecify=off  PxUpperLimitBound=1  PxUpperLimitBoundUnits=m  PxUpperLimitStiffness=1e6  PxUpperLimitStiffnessUnits=N/m  PxUpperLimitDamping=1e3  PxUpperLimitDampingUnits=N/(m/s)  PxUpperLimitTransitionRegionWidth=1e-4  PxUpperLimitTransitionRegionWidthUnits=m  PxTorqueActuationMode=NoTorque  PxMotionActuationMode=ComputedMotion  PxSensePosition=off  PxSenseVelocity=off  PxSenseAcceleration=off  PxSenseTorqueForce=off  PxSenseLowerLimitTorqueForce=off  PxSenseUpperLimitTorqueForce=off  PyPositionTargetSpecify=on  PyPositionTargetPriority=High  PyPositionTargetValue=0  PyPositionTargetValueUnits=m  PyVelocityTargetSpecify=on  PyVelocityTargetPriority=High  PyVelocityTargetValue=0  PyVelocityTargetValueUnits=m/s  PyEquilibriumPosition=0  PyEquilibriumPositionUnits=m  PySpringStiffness=SimParam.Arm.k(2,ID)  PySpringStiffnessUnits=N/m  PyDampingCoefficient=SimParam.Arm.c(2,ID)  PyDampingCoefficientUnits=N/(m/s)  PyLowerLimitSpecify=off  PyLowerLimitBound=-1  PyLowerLimitBoundUnits=m  PyLowerLimitStiffness=1e6  PyLowerLimitStiffnessUnits=N/m  PyLowerLimitDamping=1e3  PyLowerLimitDampingUnits=N/(m/s)  PyLowerLimitTransitionRegionWidth=1e-4  PyLowerLimitTransitionRegionWidthUnits=m  PyUpperLimitSpecify=off  PyUpperLimitBound=1  PyUpperLimitBoundUnits=m  PyUpperLimitStiffness=1e6  PyUpperLimitStiffnessUnits=N/m  PyUpperLimitDamping=1e3  PyUpperLimitDampingUnits=N/(m/s)  PyUpperLimitTransitionRegionWidth=1e-4  PyUpperLimitTransitionRegionWidthUnits=m  PyTorqueActuationMode=NoTorque  PyMotionActuationMode=ComputedMotion  PySensePosition=off  PySenseVelocity=off  PySenseAcceleration=off  PySenseTorqueForce=off  PySenseLowerLimitTorqueForce=off  PySenseUpperLimitTorqueForce=off  PzPositionTargetSpecify=on  PzPositionTargetPriority=High  PzPositionTargetValue=0  PzPositionTargetValueUnits=m  PzVelocityTargetSpecify=on  PzVelocityTargetPriority=High  PzVelocityTargetValue=0  PzVelocityTargetValueUnits=m/s  PzEquilibriumPosition=0  PzEquilibriumPositionUnits=m  PzSpringStiffness=SimParam.Arm.k(3,ID)  PzSpringStiffnessUnits=N/m  PzDampingCoefficient=SimParam.Arm.c(3,ID)  PzDampingCoefficientUnits=N/(m/s)  PzLowerLimitSpecify=off  PzLowerLimitBound=-1  PzLowerLimitBoundUnits=m  PzLowerLimitStiffness=1e6  PzLowerLimitStiffnessUnits=N/m  PzLowerLimitDamping=1e3  PzLowerLimitDampingUnits=N/(m/s)  PzLowerLimitTransitionRegionWidth=1e-4  PzLowerLimitTransitionRegionWidthUnits=m  PzUpperLimitSpecify=off  PzUpperLimitBound=1  PzUpperLimitBoundUnits=m  PzUpperLimitStiffness=1e6  PzUpperLimitStiffnessUnits=N/m  PzUpperLimitDamping=1e3  PzUpperLimitDampingUnits=N/(m/s)  PzUpperLimitTransitionRegionWidth=1e-4  PzUpperLimitTransitionRegionWidthUnits=m  PzTorqueActuationMode=NoTorque  PzMotionActuationMode=ComputedMotion  PzSensePosition=off  PzSenseVelocity=off  PzSenseAcceleration=off  PzSenseTorqueForce=off  PzSenseLowerLimitTorqueForce=off  PzSenseUpperLimitTorqueForce=off  SphPositionTargetSpecify=on  SphPositionTargetPriority=High  SphPositionTargetRotationMethod=AlignedAxes  SphPositionTargetFollAlignAxisA=+X  SphPositionTargetBaseAlignAxisA=+X  SphPositionTargetFollAlignAxisB=+Y  SphPositionTargetBaseAlignAxisB=+Y  SphPositionTargetRotationStandardAxis=+Z  SphPositionTargetRotationAngle=0  SphPositionTargetRotationAngleUnits=deg  SphPositionTargetRotationArbitraryAxis=[0 0 1]  SphPositionTargetRotationSequenceAxes=FollowerAxes  SphPositionTargetRotationSequence=XYX  SphPositionTargetRotationSequenceAngles=[0 0 0]  SphPositionTargetRotationSequenceAnglesUnits=deg  SphPositionTargetRotationMatrix=[1 0 0;0 1 0;0 0 1]  SphPositionTargetQuaternion=[1 0 0 0]  SphVelocityTargetSpecify=on  SphVelocityTargetPriority=High  SphVelocityTargetValue=[0 0 0]  SphVelocityTargetValueUnits=rad/s  SphVelocityTargetInFollowerFrame=on  SphEqPosRotationMethod=AlignedAxes  SphEqPosFollAlignAxisA=+X  SphEqPosBaseAlignAxisA=+X  SphEqPosFollAlignAxisB=+Y  SphEqPosBaseAlignAxisB=+Y  SphEqPosRotationStandardAxis=+Z  SphEqPosRotationAngle=0  SphEqPosRotationAngleUnits=deg  SphEqPosRotationArbitraryAxis=[0 0 1]  SphEqPosRotationSequenceAxes=FollowerAxes  SphEqPosRotationSequence=XYX  SphEqPosRotationSequenceAngles=[0 0 0]  SphEqPosRotationSequenceAnglesUnits=deg  SphEqPosRotationMatrix=[1 0 0;0 1 0;0 0 1]  SphEqPosQuaternion=[1 0 0 0]  SphSpringStiffness=SimParam.Arm.k(5,ID)  SphSpringStiffnessUnits=N*m/rad  SphDampingCoefficient=SimParam.Arm.c(5,ID)  SphDampingCoefficientUnits=N*m/(rad/s)  SphLowerLimitSpecify=off  SphLowerLimitBound=15  SphLowerLimitBoundUnits=deg  SphLowerLimitStiffness=1e4  SphLowerLimitStiffnessUnits=N*m/deg  SphLowerLimitDamping=10  SphLowerLimitDampingUnits=N*m/(deg/s)  SphLowerLimitTransitionRegionWidth=0.1  SphLowerLimitTransitionRegionWidthUnits=deg  SphUpperLimitSpecify=off  SphUpperLimitBound=45  SphUpperLimitBoundUnits=deg  SphUpperLimitStiffness=1e4  SphUpperLimitStiffnessUnits=N*m/deg  SphUpperLimitDamping=10  SphUpperLimitDampingUnits=N*m/(deg/s)  SphUpperLimitTransitionRegionWidth=0.1  SphUpperLimitTransitionRegionWidthUnits=deg  SphTorqueActuationMode=InputTorque  SphActuateTorqueX=off  SphActuateTorqueY=off  SphActuateTorqueZ=off  SphActuateTorque=off  SphActuationFrame=BaseFrame  SphSensePosition=off  SphSenseVelocityX=off  SphSenseVelocityY=off  SphSenseVelocityZ=off  SphSenseVelocity=off  SphSenseAccelerationX=off  SphSenseAccelerationY=off  SphSenseAccelerationZ=off  SphSenseAcceleration=off  SphSenseLowerLimitTorqueMag=off  SphSenseUpperLimitTorqueMag=off  SphSensingFrame=BaseFrame
  Graph : sm_lib/Frames and Transforms/Rigid Transform  RotationMethod=AlignedAxes  FollAlignAxisA=+Z  BaseAlignAxisA=+X  FollAlignAxisB=+Y  BaseAlignAxisB=+Z  RotationStandardAxis=+Z  RotationAngle=0  RotationAngleUnits=deg  RotationArbitraryAxis=[0 0 1]  RotationSequenceAxes=FollowerAxes  RotationSequence=XYX  RotationSequenceAngles=[0 0 0]  RotationSequenceAnglesUnits=deg  RotationMatrix=[1 0 0;0 1 0;0 0 1]  Quaternion=[1 0 0 0]  TranslationMethod=Cartesian  TranslationCartesianOffset=[(SimParam.Arm.l(1,ID)+SimParam.Arm.l(2,ID))/2 0 0]  TranslationCartesianOffsetUnits=m  TranslationStandardAxis=+Z  TranslationStandardOffset=0  TranslationStandardOffsetUnits=m  TranslationROffset=0  TranslationROffsetUnits=m  TranslationThetaOffset=0  TranslationThetaOffsetUnits=deg  TranslationZOffset=0  TranslationZOffsetUnits=m
  Graph only : sm_lib/Body Elements/Extruded Solid  ExtrusionType=General  PolygonNumSides=3  PolygonOuterRadius=1  PolygonOuterRadiusUnits=m  ExportEntireGeometry=off  ExtrusionCrossSection=0.01.*[1 1; -1 1; -1 -1; 1 -1]  ExtrusionCrossSectionUnits=m  ExportConvexHullGeometry=off  ExtrusionLength=SimParam.Arm.l(1,ID)+SimParam.Arm.l(2,ID)  ExtrusionLengthUnits=m  InertiaType=PointMass  BasedOnType=Density  Density=1000  DensityUnits=kg/(m^3)  Mass=0  MassUnits=kg  CenterOfMass=[0 0 0]  CenterOfMassUnits=m  MomentsOfInertia=[0 0 0]  MomentsOfInertiaUnits=kg*m^2  ProductsOfInertia=[0 0 0]  ProductsOfInertiaUnits=kg*m^2  GraphicType=FromGeometry  MarkerShape=Sphere  MarkerSize=10  GraphicVisPropType=SimpleVisualProperties  GraphicDiffuseColor=[0.5 0.5 0.5]  GraphicOpacity=1.0  GraphicSpecularColor=[0.5 0.5 0.5 1.0]  GraphicAmbientColor=[0.15 0.15 0.15 1.0]  GraphicEmissiveColor=[0.0 0.0 0.0 1.0]  GraphicShininess=75  DoExposeReferenceFrame=on  SerializedFrames=<Frames/>
  Inertia : sm_lib/Body Elements/Inertia  InertiaType=Custom  Mass=SimParam.Arm.m(ID)  MassUnits=kg  CenterOfMass=[0 0 0]  CenterOfMassUnits=m  MomentsOfInertia=SimParam.Arm.I(:,ID)'  MomentsOfInertiaUnits=kg*m^2  ProductsOfInertia=[0 0 0]  ProductsOfInertiaUnits=kg*m^2  GraphicType=Marker  MarkerShape=Inertia  MarkerSize=20  GraphicVisPropType=SimpleVisualProperties  GraphicDiffuseColor=[0.5 0.5 0.5]  GraphicOpacity=1  GraphicSpecularColor=[0.5 0.5 0.5 1.0]  GraphicAmbientColor=[0.15 0.15 0.15 1.0]  GraphicEmissiveColor=[0.0 0.0 0.0 1.0]  GraphicShininess=75
  Rigid Transform : sm_lib/Frames and Transforms/Rigid Transform  RotationMethod=None  FollAlignAxisA=+X  BaseAlignAxisA=+Y  FollAlignAxisB=+Y  BaseAlignAxisB=+Z  RotationStandardAxis=+Z  RotationAngle=0  RotationAngleUnits=deg  RotationArbitraryAxis=[0 0 1]  RotationSequenceAxes=FollowerAxes  RotationSequence=XYX  RotationSequenceAngles=[0 0 0]  RotationSequenceAnglesUnits=deg  RotationMatrix=[1 0 0;0 1 0;0 0 1]  Quaternion=[1 0 0 0]  TranslationMethod=Cartesian  TranslationCartesianOffset=[SimParam.Arm.l(1,ID) 0 0]  TranslationCartesianOffsetUnits=m  TranslationStandardAxis=+Z  TranslationStandardOffset=0  TranslationStandardOffsetUnits=m  TranslationROffset=0  TranslationROffsetUnits=m  TranslationThetaOffset=0  TranslationThetaOffsetUnits=deg  TranslationZOffset=0  TranslationZOffsetUnits=m
  Rigid Transform1 : sm_lib/Frames and Transforms/Rigid Transform  RotationMethod=None  FollAlignAxisA=+X  BaseAlignAxisA=+Y  FollAlignAxisB=+Y  BaseAlignAxisB=+Z  RotationStandardAxis=+Z  RotationAngle=0  RotationAngleUnits=deg  RotationArbitraryAxis=[0 0 1]  RotationSequenceAxes=FollowerAxes  RotationSequence=XYX  RotationSequenceAngles=[0 0 0]  RotationSequenceAnglesUnits=deg  RotationMatrix=[1 0 0;0 1 0;0 0 1]  Quaternion=[1 0 0 0]  TranslationMethod=Cartesian  TranslationCartesianOffset=[SimParam.Arm.l(2,ID) 0 0]  TranslationCartesianOffsetUnits=m  TranslationStandardAxis=+Z  TranslationStandardOffset=0  TranslationStandardOffsetUnits=m  TranslationROffset=0  TranslationROffsetUnits=m  TranslationThetaOffset=0  TranslationThetaOffsetUnits=deg  TranslationZOffset=0  TranslationZOffsetUnits=m
  in : PMIOPort  Side=Left
  out : PMIOPort  Port=2  Side=Right
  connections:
  Rigid Transform/RConn1 -- Rigid Transform1/LConn1 -- Inertia/RConn1
  Rigid Transform/LConn1 -- 6-DOF Joint/RConn1 -- Graph/LConn1
  Rigid Transform1/RConn1 -- out/RConn1
  Graph only/RConn1 -- Graph/RConn1
  6-DOF Joint/LConn1 -- in/RConn1

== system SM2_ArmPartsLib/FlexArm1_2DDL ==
  FirstSegment : $bdroot/ArmFirstSegment  ID=1
  Segment : $bdroot/ArmSegment  ID=2
  Motor : PMIOPort  Side=Left
  ForeArm : PMIOPort  Port=2  Side=Right
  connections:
  FirstSegment/LConn1 -- Motor/RConn1
  FirstSegment/RConn1 -- Segment/LConn1
  ForeArm/RConn1 -- Segment/RConn1

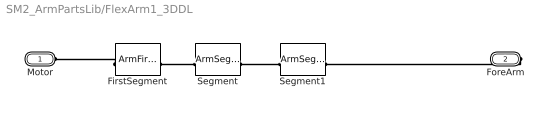
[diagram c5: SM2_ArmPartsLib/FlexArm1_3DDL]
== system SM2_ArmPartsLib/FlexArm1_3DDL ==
  FirstSegment : $bdroot/ArmFirstSegment  ID=1
  Segment : $bdroot/ArmSegment  ID=2
  Segment1 : $bdroot/ArmSegment  ID=3
  Motor : PMIOPort  Side=Left
  ForeArm : PMIOPort  Port=2  Side=Right
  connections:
  FirstSegment/LConn1 -- Motor/RConn1
  FirstSegment/RConn1 -- Segment/LConn1
  Segment/RConn1 -- Segment1/LConn1
  ForeArm/RConn1 -- Segment1/RConn1

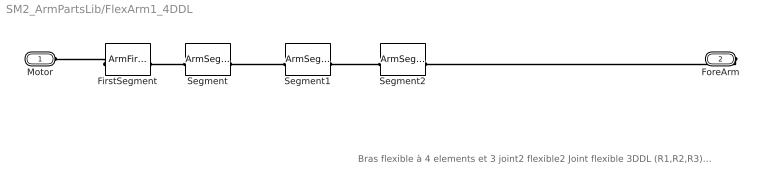
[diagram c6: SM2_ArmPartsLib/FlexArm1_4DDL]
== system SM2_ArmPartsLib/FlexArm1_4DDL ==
  note: Bras flexible à 4 elements et 3 joint2 flexible2 Joint flexible 3DDL (R1,R2,R3) coordonnees : x : Aligne avec axe du bras y : Tjs dans le plan horizontal (Xw,Yw) z : x^y Parametres du segments n°ID Solid Longeurs debut-cg : ArmParam.l(1,ID) Longueur cg-fin : ArmParam.l(2,ID) Masse cg : ArmParam.m(ID) Inertie cg : ArmParam.I(:,ID)' Rigid transforms Longueur debut-cg : ArmParam.l(1,ID) Longueur cg-fin : ArmParam.l(2,ID) Joint Rigidite : ArmParam.k(1..3,ID) Amortissement : ArmParam.c(1..3,ID)
  FirstSegment : $bdroot/ArmFirstSegment  ID=1
  Segment : $bdroot/ArmSegment  ID=2
  Segment1 : $bdroot/ArmSegment  ID=3
  Segment2 : $bdroot/ArmSegment  ID=4
  Motor : PMIOPort  Side=Left
  ForeArm : PMIOPort  Port=2  Side=Right
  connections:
  FirstSegment/LConn1 -- Motor/RConn1
  FirstSegment/RConn1 -- Segment/LConn1
  Segment1/LConn1 -- Segment/RConn1
  Segment1/RConn1 -- Segment2/LConn1
  ForeArm/RConn1 -- Segment2/RConn1

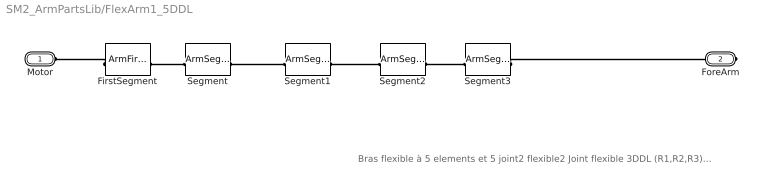
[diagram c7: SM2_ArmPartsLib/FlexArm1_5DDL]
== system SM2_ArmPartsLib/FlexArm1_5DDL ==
  note: Bras flexible à 5 elements et 5 joint2 flexible2 Joint flexible 3DDL (R1,R2,R3) coordonnees : x : Aligne avec axe du bras y : Tjs dans le plan horizontal (Xw,Yw) z : x^y Parametres du segments n°ID Solid Longeurs debut-cg : ArmParam.l(1,ID) Longueur cg-fin : ArmParam.l(2,ID) Masse cg : ArmParam.m(ID) Inertie cg : ArmParam.I(:,ID)' Rigid transforms Longueur debut-cg : ArmParam.l(1,ID) Longueur cg-fin : ArmParam.l(2,ID) Joint Rigidite : ArmParam.k(1..3,ID) Amortissement : ArmParam.c(1..3,ID)
  FirstSegment : $bdroot/ArmFirstSegment  ID=1
  Segment : $bdroot/ArmSegment  ID=2
  Segment1 : $bdroot/ArmSegment  ID=3
  Segment2 : $bdroot/ArmSegment  ID=4
  Segment3 : $bdroot/ArmSegment  ID=5
  Motor : PMIOPort  Side=Left
  ForeArm : PMIOPort  Port=2  Side=Right
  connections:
  FirstSegment/LConn1 -- Motor/RConn1
  FirstSegment/RConn1 -- Segment/LConn1
  Segment1/LConn1 -- Segment/RConn1
  Segment1/RConn1 -- Segment2/LConn1
  Segment3/LConn1 -- Segment2/RConn1
  Segment3/RConn1 -- ForeArm/RConn1

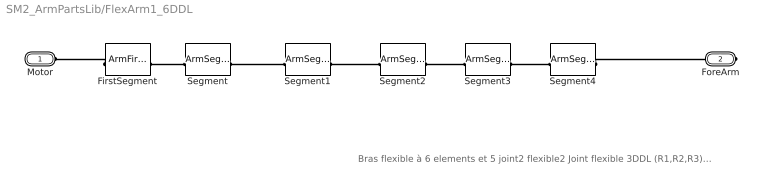
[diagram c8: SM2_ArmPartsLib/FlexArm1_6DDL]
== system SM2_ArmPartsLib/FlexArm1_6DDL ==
  note: Bras flexible à 6 elements et 5 joint2 flexible2 Joint flexible 3DDL (R1,R2,R3) coordonnees : x : Aligne avec axe du bras y : Tjs dans le plan horizontal (Xw,Yw) z : x^y Parametres du segments n°ID Solid Longeurs debut-cg : ArmParam.l(1,ID) Longueur cg-fin : ArmParam.l(2,ID) Masse cg : ArmParam.m(ID) Inertie cg : ArmParam.I(:,ID)' Rigid transforms Longueur debut-cg : ArmParam.l(1,ID) Longueur cg-fin : ArmParam.l(2,ID) Joint Rigidite : ArmParam.k(1..3,ID) Amortissement : ArmParam.c(1..3,ID)
  FirstSegment : $bdroot/ArmFirstSegment  ID=1
  Segment : $bdroot/ArmSegment  ID=2
  Segment1 : $bdroot/ArmSegment  ID=3
  Segment2 : $bdroot/ArmSegment  ID=4
  Segment3 : $bdroot/ArmSegment  ID=5
  Segment4 : $bdroot/ArmSegment  ID=6
  Motor : PMIOPort  Side=Left
  ForeArm : PMIOPort  Port=2  Side=Right
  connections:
  FirstSegment/LConn1 -- Motor/RConn1
  FirstSegment/RConn1 -- Segment/LConn1
  Segment1/LConn1 -- Segment/RConn1
  Segment1/RConn1 -- Segment2/LConn1
  Segment3/LConn1 -- Segment2/RConn1
  Segment3/RConn1 -- Segment4/LConn1
  Segment4/RConn1 -- ForeArm/RConn1

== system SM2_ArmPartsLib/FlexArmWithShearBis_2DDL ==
  ArmSegmentWithShearbis : $bdroot/ArmSegmentWithShearbis  ID=1
  ArmSegmentWithShearbis1 : $bdroot/ArmSegmentWithShearbis  ID=2
  Motor : PMIOPort  Side=Left
  ForeArm : PMIOPort  Port=2  Side=Right
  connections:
  ArmSegmentWithShearbis/LConn1 -- Motor/RConn1
  ArmSegmentWithShearbis1/LConn1 -- ArmSegmentWithShearbis/RConn1
  ArmSegmentWithShearbis1/RConn1 -- ForeArm/RConn1

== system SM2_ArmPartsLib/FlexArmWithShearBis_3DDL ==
  ArmSegmentWithShearbis : $bdroot/ArmSegmentWithShearbis  ID=1
  ArmSegmentWithShearbis1 : $bdroot/ArmSegmentWithShearbis  ID=2
  ArmSegmentWithShearbis2 : $bdroot/ArmSegmentWithShearbis  ID=3
  Motor : PMIOPort  Side=Left
  ForeArm : PMIOPort  Port=2  Side=Right
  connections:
  ArmSegmentWithShearbis/LConn1 -- Motor/RConn1
  ArmSegmentWithShearbis1/LConn1 -- ArmSegmentWithShearbis/RConn1
  ForeArm/RConn1 -- ArmSegmentWithShearbis2/RConn1
  ArmSegmentWithShearbis2/LConn1 -- ArmSegmentWithShearbis1/RConn1

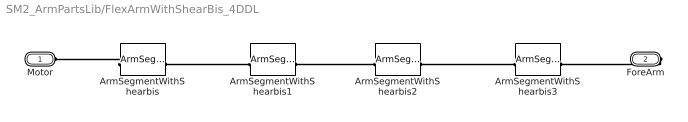
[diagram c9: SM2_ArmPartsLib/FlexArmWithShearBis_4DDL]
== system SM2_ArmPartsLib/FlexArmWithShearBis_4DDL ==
  ArmSegmentWithShearbis : $bdroot/ArmSegmentWithShearbis  ID=1
  ArmSegmentWithShearbis1 : $bdroot/ArmSegmentWithShearbis  ID=2
  ArmSegmentWithShearbis2 : $bdroot/ArmSegmentWithShearbis  ID=3
  ArmSegmentWithShearbis3 : $bdroot/ArmSegmentWithShearbis  ID=4
  Motor : PMIOPort  Side=Left
  ForeArm : PMIOPort  Port=2  Side=Right
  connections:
  ArmSegmentWithShearbis/LConn1 -- Motor/RConn1
  ArmSegmentWithShearbis1/LConn1 -- ArmSegmentWithShearbis/RConn1
  ArmSegmentWithShearbis2/LConn1 -- ArmSegmentWithShearbis1/RConn1
  ForeArm/RConn1 -- ArmSegmentWithShearbis3/RConn1
  ArmSegmentWithShearbis3/LConn1 -- ArmSegmentWithShearbis2/RConn1

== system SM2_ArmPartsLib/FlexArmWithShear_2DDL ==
  ArmSegmentWithShear : $bdroot/ArmSegmentWithShear  ID=1
  ArmSegmentWithShear1 : $bdroot/ArmSegmentWithShear  ID=2
  Motor : PMIOPort  Side=Left
  ForeArm : PMIOPort  Port=2  Side=Right
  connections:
  ArmSegmentWithShear/LConn1 -- Motor/RConn1
  ArmSegmentWithShear1/LConn1 -- ArmSegmentWithShear/RConn1
  ArmSegmentWithShear1/RConn1 -- ForeArm/RConn1

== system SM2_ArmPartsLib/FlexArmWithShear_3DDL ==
  ArmSegmentWithShear : $bdroot/ArmSegmentWithShear  ID=1
  ArmSegmentWithShear1 : $bdroot/ArmSegmentWithShear  ID=2
  ArmSegmentWithShear2 : $bdroot/ArmSegmentWithShear  ID=3
  Motor : PMIOPort  Side=Left
  ForeArm : PMIOPort  Port=2  Side=Right
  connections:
  ArmSegmentWithShear/LConn1 -- Motor/RConn1
  ArmSegmentWithShear1/LConn1 -- ArmSegmentWithShear/RConn1
  ForeArm/RConn1 -- ArmSegmentWithShear2/RConn1
  ArmSegmentWithShear2/LConn1 -- ArmSegmentWithShear1/RConn1

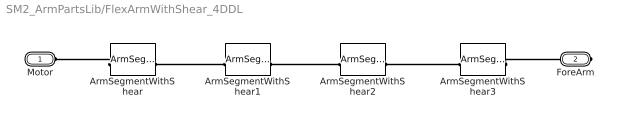
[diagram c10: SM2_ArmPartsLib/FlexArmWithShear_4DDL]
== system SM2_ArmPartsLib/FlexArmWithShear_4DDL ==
  ArmSegmentWithShear : $bdroot/ArmSegmentWithShear  ID=1
  ArmSegmentWithShear1 : $bdroot/ArmSegmentWithShear  ID=2
  ArmSegmentWithShear2 : $bdroot/ArmSegmentWithShear  ID=3
  ArmSegmentWithShear3 : $bdroot/ArmSegmentWithShear  ID=4
  Motor : PMIOPort  Side=Left
  ForeArm : PMIOPort  Port=2  Side=Right
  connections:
  ArmSegmentWithShear/LConn1 -- Motor/RConn1
  ArmSegmentWithShear1/LConn1 -- ArmSegmentWithShear/RConn1
  ArmSegmentWithShear1/RConn1 -- ArmSegmentWithShear2/LConn1
  ArmSegmentWithShear2/RConn1 -- ArmSegmentWithShear3/LConn1
  ArmSegmentWithShear3/RConn1 -- ForeArm/RConn1
